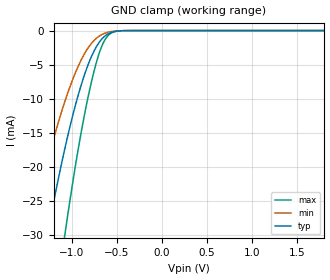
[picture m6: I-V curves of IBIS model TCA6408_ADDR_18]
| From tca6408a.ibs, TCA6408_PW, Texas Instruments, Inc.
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[Model]   TCA6408_ADDR_18
Model_type  Input
Vinl=0.495
Vinh=1.365
| variable   typ   min   max
C_comp   2.22pF   1.67pF   2.46pF
[Temperature Range]   40   100   -40
| Ambient temperature   25   85   -40
[Voltage range]   1.8   1.65   1.95
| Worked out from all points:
|   GND clamp passes 1 mA (typ) near -0.65 V on its own axis
[GND Clamp]
| TCA6408_ADDR_18
|   Voltage   I(typ)   I(min)   I(max)
-1.8V     -74.02mA   -51.67mA   -111.7mA
-1.45V    -43.77mA   -29.21mA   -69.33mA
-1.27V    -30.12mA   -19.36mA   -49.42mA
-1.25V    -28.7mA    -18.35mA   -47.31mA
-1.07V    -17.07mA   -10.25mA   -29.6mA
-960mV    -11.11mA   -6.281mA   -20.1mA
-855mV    -6.438mA   -3.375mA   -12.27mA
-765mV    -3.406mA   -1.667mA   -6.757mA
-680mV    -1.498mA   -708.4uA   -2.836mA
-590mV    -450.5uA   -228.8uA   -677.8uA
-475mV    -54.97uA   -37.86uA   -56.06uA
1.8V      147.6pA    546pA      30.99pA
